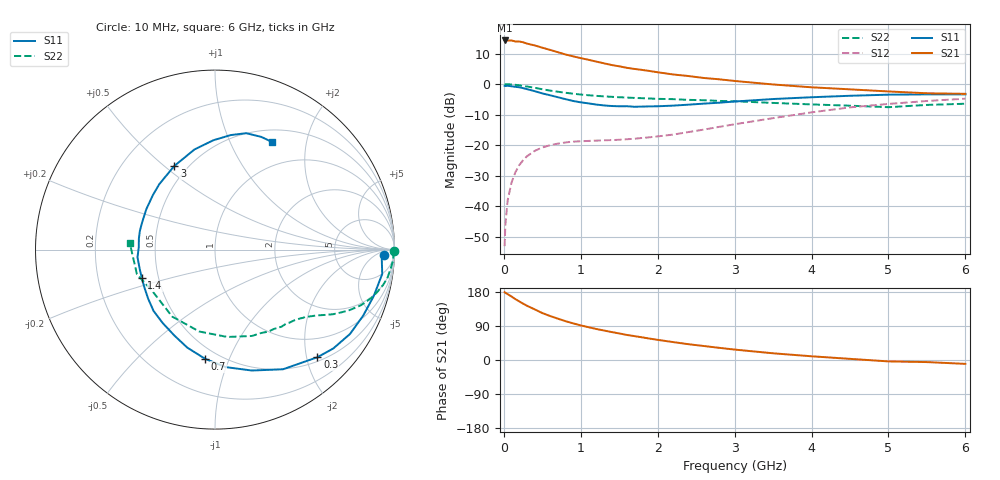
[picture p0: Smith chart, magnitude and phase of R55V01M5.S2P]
! SIEMENS Small Signal Semiconductors
! BFR183
! Si NPN RF Bipolar Junction Transistor in SOT23
! VCE = 5 V  IC = 1.5 mA
! Common Emitter S-Parameters:  May  1996
# GHz  S  MA  R  50
!  f  S11  S21  S12  S22
! GHz  MAG  ANG  MAG  ANG  MAG  ANG  MAG  ANG
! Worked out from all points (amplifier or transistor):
!   36 points, 10 MHz to 6 GHz, reference 50 ohm
!   highest |S21| = 14.3 dB at 10 MHz (marker M1)
!   |S21| within 3 dB of that: start of sweep to 587.8 MHz
!   unconditionally stable (mu >= 1): 1.509 GHz to 2.88 GHz
!   at 250 MHz: K = 0.19, MSG = 19.3 dB, |S12| = -25.0 dB
!   at 1.4 GHz: K = 0.96, MSG = 12.3 dB, |S12| = -18.4 dB
!   at 6 GHz: K = 0.92, MSG = 0.8 dB, |S12| = -4.8 dB
!   S11 on the Smith chart (normalised r, x): 10 MHz: 26, -12; 300 MHz: 0.58, -2.21; 700 MHz: 0.42, -0.82; 1.4 GHz: 0.40, -0.16; 3 GHz: 0.42, +0.54; 6 GHz: 0.65, +1.45
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0.01  0.9395 -1.7  5.201 179.1  0.0022 92.1  0.9973 -0.6
0.02  0.9308 -3.3  5.091 177.4  0.0049 83.8  0.9935 -1.2
0.05  0.9415 -8.3  5.171 173.7  0.0125 86.4  0.9947 -3.2
0.1  0.9215 -16.3  5.197 167.5  0.0243 80.6  0.9845 -6.2
0.15  0.9039 -24.0  5.007 160.6  0.0359 75.8  0.9735 -9.3
0.2  0.887 -32.0  4.995 154.7  0.0468 71.7  0.957 -11.9
0.25  0.8589 -39.9  4.861 148.7  0.0565 67.6  0.9348 -14.6
0.3  0.8278 -46.4  4.622 143.2  0.0655 64.2  0.9137 -17.0
0.4  0.7669 -60.4  4.316 133.7  0.0803 57.5  0.8712 -20.8
0.5  0.7041 -73.1  3.959 123.9  0.0913 51.8  0.8238 -24.1
0.6  0.6571 -84.9  3.645 116.2  0.0994 47.5  0.7831 -26.6
0.7  0.6108 -95.2  3.344 109.2  0.1056 44.3  0.7514 -28.6
0.9  0.5293 -115.4  2.857 96.7  0.114 39.9  0.6968 -31.6
1.1  0.4836 -135.1  2.509 86.6  0.1171 38.4  0.657 -34.3
1.4  0.4375 -158.7  2.059 73.8  0.1206 38.9  0.6195 -37.9
1.8  0.4284 171.9  1.708 59.7  0.131 44.2  0.5879 -42.7
2.2  0.4439 149.6  1.44 47.3  0.1487 50.3  0.5671 -49.3
3  0.518 116.0  1.127 27.5  0.2196 55.6  0.5235 -66.8
3.5  0.5695 101.6  0.987 17.7  0.2768 53.2  0.4917 -81.9
4.5  0.644 82.2  0.821 3.0  0.4157 41.3  0.4428 -122.6
5.5  0.6788 67.7  0.708 -5.5  0.5291 25.8  0.4561 -162.5
6  0.6786 62.3  0.693 -10.2  0.5765 16.2  0.4767 175.4
